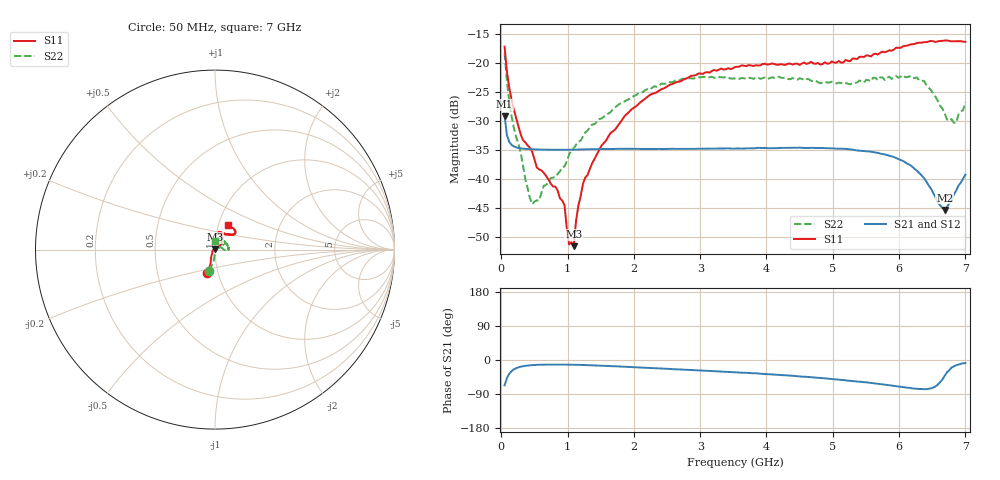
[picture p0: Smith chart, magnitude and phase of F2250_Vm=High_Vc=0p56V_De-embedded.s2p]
! Integrated Device Technology
! Corporate Headquarters
! 6024 Silver Creek Valley Road
! San Jose, CA 95138  USA
! Phone:  1-408-284-8200
! Toll Free:  1-800-223-1366
! Webpage:  http://www.idt.com/
! Timing and RF Division
! 515 Groton Road, Suite 102
! Westford, MA 01886-6024
! Device:  F2250
! Description: Voltage Variable RF Attenuator
! Frequency:  50.0 -  6000.00 MHz
! Package:  3x3 mm Thin QFN Plastic Package: 16 pin
! Ports:  2 RF, 3 DC
!  Pin  1  = GND
!  Pin  2  = NC
!  Pin  3  = RF1  = Port 1
!  Pin  4  = NC
!  Pin  5  = GND
!  Pin  6  = GND
!  Pin  7  = GND
!  Pin  8  = GND
!  Pin  9  = NC
!  Pin 10  = RF2  = Port 2
!  Pin 11  = NC
!  Pin 12  = GND
!  Pin 13  = GND
!  Pin 14  = VCNTRL
!  Pin 15  = VDD
!  Pin 16  = VMODE
! Vcntrl:  0.560 Volts
! Vmode:  +3.300 Volts
! Vdd:  +3.30  Volts
! Current:  1.269 mA
! Data:  The device was measured on a the F2250 evaluation board which has
!  individual transmission lines to the RF pins.  Data was collected
!  using a calibrated network analyzer.  The evaluation board was
!  de-embedded using a TRL calibration technique.
!  The reference plane is the edge of the package pin.
! Misc:  SN 10
!  Action Tracker AT0258
! Date Measured:  2014-11-26
! Date:  2015-10-15  MJV
! Note:
!  Integrated Device Technology supplies this data as a sample of measured
!  data at the package pin for this product.  Your particular data for this
!  product may vary.
!  Data was taken at 25 degrees C.
!  Integrated Device Technology reserves the right to change this data at anytime.
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# GHz S dB R 50
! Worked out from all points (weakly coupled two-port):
!   201 points, 50 MHz to 7 GHz, reference 50 ohm
!   highest |S21| = -29.12 dB at 50 MHz (marker M1); lowest = -45.3 dB at 6.687 GHz (marker M2)
!   lowest |S11| = -51.5 dB at 1.093 GHz (marker M3), VSWR 1.01, Z = 50 + j0.266 ohm
!   |S11| at or under -10 dB: start of sweep to end of sweep
!   |S22| runs from -44.3 to -18.3 dB; largest |S21 - S12| = 5e-05
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0.05  -17.17 -108.4  -29.12 -66.7  -29.12 -66.7  -18.28 -105.7
0.08475  -21.46 -107.3  -32.38 -47.6  -32.38 -47.6  -23.06 -96.9
0.189  -28.01 -119.7  -34.33 -24.9  -34.33 -24.9  -31.12 -92.0
0.328  -33.27 -133.7  -34.72 -16.4  -34.72 -16.4  -37.73 -68.8
0.467  -35.29 -145.8  -34.83 -13.5  -34.83 -13.5  -44.28 -38.7
0.5365  -37.97 -154.1  -34.86 -12.8  -34.86 -12.8  -43.63 -19.5
0.64075  -38.88 -162.3  -34.88 -12.2  -34.89 -12.2  -41.11 5.0
0.8145  -41.24 169.9  -34.91 -12.0  -34.91 -12.0  -39.60 20.9
0.9535  -44.46 171.0  -34.91 -12.1  -34.92 -12.2  -37.78 25.1
1.023  -51.21 139.4  -34.90 -12.3  -34.90 -12.3  -35.73 24.7
1.0925  -51.50 86.8  -34.88 -12.5  -34.89 -12.5  -34.68 26.4
1.12725  -47.18 59.5  -34.88 -12.7  -34.88 -12.7  -34.03 23.8
1.2315  -40.78 39.8  -34.85 -13.1  -34.85 -13.1  -32.63 21.4
1.6485  -32.00 40.9  -34.78 -16.1  -34.78 -16.1  -28.43 29.1
2.37825  -24.75 46.5  -34.76 -22.2  -34.76 -22.3  -23.89 36.3
3.525  -20.66 71.6  -34.71 -32.4  -34.71 -32.5  -22.64 62.6
4.7065  -20.07 71.9  -34.59 -46.0  -34.59 -46.0  -23.08 64.0
5.85325  -17.80 40.5  -35.95 -66.6  -35.96 -66.7  -22.33 13.6
6.3745  -16.41 40.9  -39.76 -77.0  -39.77 -77.1  -23.05 -3.0
6.68725  -16.12 47.8  -45.26 -41.8  -45.25 -41.7  -28.60 19.0
6.861  -16.22 54.4  -41.92 -13.9  -41.90 -13.9  -30.28 59.5
7  -16.33 62.4  -39.20 -8.2  -39.17 -8.3  -26.76 92.3
